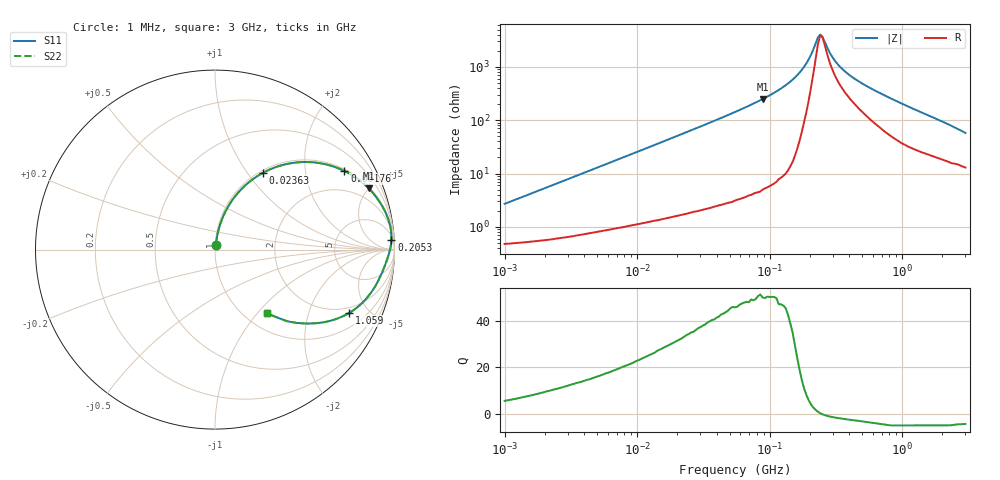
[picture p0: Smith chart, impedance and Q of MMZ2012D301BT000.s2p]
! S-parameter Generated by TDK Corporation
! Copyright(C) 2016 TDK Corporation.
! All Rights Reserved.
! TDK P/N: MMZ2012D301BT000 (Chip Beads)
! Property: |Z|=300¶ at 100MHz
! Size(LxWxT): 2x1.25x0.85mm, 0.079x0.049x0.033inches
! Model Type: s2p (Touchstone File Format Version 1.0)
! Frequency: DC=Yes Start=1MHz Stop=3000MHz 202points Log-sweep
! Note: This model was converted from impedance.
! Model Generated on May. 16, 2016
! Hash(MD5):
! Port Assignments:
!  1 ---@@@--- 2
! Applicable Conditions:
!  Temperature = 25 degC
!  DC Bias Current = 0 A
!  Small Signal Operation
! Terms and conditions regarding TDK Simulation Models
! (1)This simulation model is being provided solely for informational purposes. Please refer to the specifications of the products in terms of detailed characteristics of such products.
! (2)In no event shall TDK Corporation of any of its subsidiaries be liable for any loss or damage arising, directly or indirectly,
!  From any information contained in this simulation model, including, but not limited to loss or damages arising from any inaccuracies, omissions or errors in connection with such information.
! (3)Any and all copyrights on this simulation model are owned by TDK Corporation.
!  Duplication or redistribution of this simulation model without prior written permission from TDK Corporation is prohibited.
! (4)This simulation model is subject to any modification or change without any prior notice.
! (5)Neither TDK Corporation nor any of its subsidiaries shall make any warranty, express or implied,
!  Including but not limited to the correctness, implied warranties of merchantability and fitness for a particular purpose with respect to this simulation models.
! (6)The use of this simulation model shall be deemed to have consented to the terms and conditions hereof.
# MHz S MA R 50
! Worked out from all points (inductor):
!   201 points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, 1 MHz to 3 GHz, reference 50 ohm
!   read as one part in series: L = 421 nH near 1.041 MHz
!   highest Q = 50.3 at 88.55 MHz (marker M1), where L = 448 nH
!   self-resonance near 240.9 MHz
!   S11 on the Smith chart (normalised r, x): 1 MHz: 1.01, +0.05; 23.63 MHz: 1.04, +1.19; 61.76 MHz: 1.07, +3.25; 205.3 MHz: 9, +33; 1.059 GHz: 1.68, -3.74; 3 GHz: 1.26, -1.12
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1  0.02685 78.3  0.9949 -1.5  0.9949 -1.5  0.02685 78.3
3.900413  0.1 80.2  0.9879 -5.7  0.9879 -5.7  0.1 80.2
14.61624  0.3427 67.9  0.9271 -20.0  0.9271 -20.0  0.3427 67.9
23.62996  0.5056 57.9  0.8479 -30.4  0.8479 -30.4  0.5056 57.9
36.70325  0.6738 46.2  0.7224 -42.3  0.7224 -42.3  0.6738 46.2
54.77226  0.81 34.7  0.5691 -54.1  0.5691 -54.1  0.81 34.7
61.76144  0.8437 31.3  0.5193 -57.5  0.5193 -57.5  0.8437 31.3
88.54986  0.9216 21.7  0.3701 -67.1  0.3701 -67.1  0.9216 21.7
149.005  0.9805 9.8  0.1703 -78.6  0.1703 -78.6  0.9805 9.8
174.8812  0.986 6.4  0.1124 -79.6  0.1124 -79.6  0.986 6.4
205.2512  0.9842 3.2  0.05836 -72.7  0.05836 -72.7  0.9842 3.2
213.6344  0.9828 2.5  0.04638 -67.0  0.04638 -67.0  0.9828 2.5
231.4421  0.9791 1.0  0.02752 -40.1  0.02752 -40.1  0.9791 1.0
240.8952  0.9766 0.3  0.02413 -13.8  0.02413 -13.8  0.9766 0.3
250.7343  0.9739 -0.3  0.02672 11.7  0.02672 11.7  0.9739 -0.3
294.2768  0.9627 -2.8  0.06058 50.6  0.06058 50.6  0.9627 -2.8
359.4878  0.9495 -5.6  0.1085 59.5  0.1085 59.5  0.9495 -5.6
495.1867  0.9278 -10.4  0.1883 62.4  0.1883 62.4  0.9278 -10.4
800.5644  0.8785 -19.1  0.3332 59.4  0.3332 59.4  0.8785 -19.1
1059.487  0.8264 -25.3  0.4344 54.4  0.4344 54.4  0.8264 -25.3
1855.641  0.6572 -38.8  0.6385 40.2  0.6385 40.2  0.6572 -38.8
3000  0.4573 -50.6  0.7925 26.5  0.7925 26.5  0.4573 -50.6
